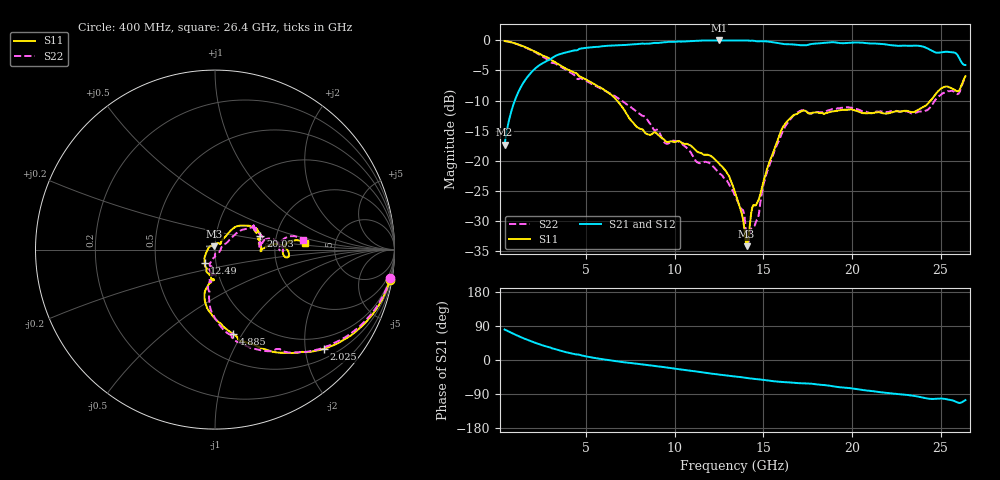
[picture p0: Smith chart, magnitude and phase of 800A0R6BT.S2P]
!  American Technical Ceramics  Date:  12/17/08
!  One Norden Lane
!  Huntington Station,  NY.  11746-2102
!  Tel:  (631) 622-4700  Fax:  (631) 622-4748
!  Part Number  800A0R6BT
!  Description: Broardband capacitor  Mounting Orientation: Vertical
!  Application:
# GHZ S DB R 50
! Freq  |S11|  S11 Ph  |S21|  S21 Ph  |S12|  S12 Ph  |S22|  S22 Ph
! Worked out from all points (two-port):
!   401 points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, 400 MHz to 26.4 GHz, reference 50 ohm
!   highest |S21| = 0.00 dB at 12.49 GHz (marker M1); lowest = -17.3 dB at 400 MHz (marker M2)
!   |S21| within 3 dB of the highest: 3.049 GHz to 26.06 GHz (23.02 GHz wide, 158 % of centre)
!   lowest |S11| = -34.2 dB at 14.05 GHz (marker M3), VSWR 1.04, Z = 49.5 + j1.88 ohm
!   |S11| at or under -10 dB: 6.743 GHz to 24.44 GHz (17.7 GHz wide, 114 % of centre)
!   |S22| runs from -34.2 to -0.1 dB; largest |S21 - S12| = 0.0038
!   S11 on the Smith chart (normalised r, x): 400 MHz: 1, -12; 2.025 GHz: 0.71, -2.40; 4.885 GHz: 0.75, -0.92; 12.49 GHz: 0.88, -0.13; 20.03 GHz: 1.65, +0.27; 26.4 GHz: 2.99, +0.32
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0.4  -0.09 -9.7  -17.34 80.4  -17.36 80.4  -0.09 -9.1
1.05  -0.55 -24.5  -9.44 65.8  -9.45 65.8  -0.56 -23.2
2.025  -1.72 -42.4  -4.95 47.2  -4.96 47.2  -1.81 -42.4
4.755  -6.15 -76.6  -1.32 11.9  -1.33 12.0  -6.35 -79.9
4.885  -6.35 -77.8  -1.27 10.5  -1.28 10.6  -6.55 -81.5
6.9  -10.55 -100.7  -0.77 -4.5  -0.77 -4.4  -9.81 -94.8
7.875  -14.44 -98.8  -0.61 -9.9  -0.60 -9.8  -11.91 -97.4
9.11  -15.85 -97.7  -0.41 -17.1  -0.40 -17.0  -15.17 -99.6
12.49  -20.44 -127.2  0.00 -38.3  -0.01 -38.2  -22.03 -109.6
13.4  -25.27 -157.1  -0.01 -43.5  -0.01 -43.5  -25.90 -103.2
14.05  -34.24 102.6  -0.01 -47.5  -0.01 -47.5  -33.28 -82.6
14.635  -27.16 46.7  -0.13 -50.7  -0.12 -50.7  -29.83 0.9
15.155  -21.94 52.1  -0.15 -53.4  -0.14 -53.4  -22.40 30.2
16.065  -14.62 45.3  -0.56 -58.0  -0.55 -58.0  -15.32 37.1
16.91  -12.21 30.6  -0.73 -60.9  -0.71 -60.9  -12.00 29.2
17.755  -12.05 23.9  -0.57 -62.9  -0.55 -62.9  -12.11 29.6
20.03  -11.54 17.0  -0.36 -75.1  -0.34 -75.1  -11.25 10.0
22.11  -12.09 6.8  -0.76 -87.9  -0.74 -88.0  -11.85 8.7
24.19  -10.78 3.6  -1.22 -101.2  -1.20 -101.3  -11.67 8.0
25.165  -7.77 -1.5  -1.92 -102.2  -1.91 -102.3  -8.75 4.5
26.01  -8.43 0.8  -2.69 -112.9  -2.68 -113.0  -8.88 4.6
26.4  -5.97 4.5  -4.09 -105.9  -4.07 -106.0  -6.09 6.5
